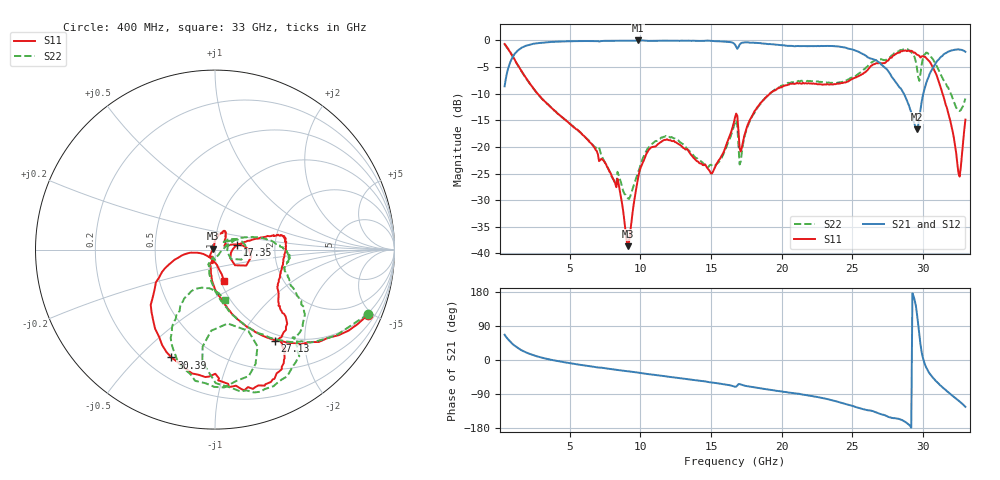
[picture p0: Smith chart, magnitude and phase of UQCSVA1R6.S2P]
!  Part Number  UQCSVA1R6  Mounting Orientation: Horizontal
!  Description: Ultra Low ESR Microwave capacitors
!  Application: Coupling, Bypass, Tuning, DC Block
!  Filters, Matching
# GHZ S DB R 50
! Freq  |S11|  S11 Ph  |S21|  S21 Ph  |S12|  S12 Ph  |S22|  S22 Ph
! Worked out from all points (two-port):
!   401 points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, 400 MHz to 33 GHz, reference 50 ohm
!   highest |S21| = 0.00 dB at 9.854 GHz (marker M1); lowest = -16.7 dB at 29.58 GHz (marker M2)
!   |S21| within 3 dB of the highest: 1 GHz to 26.02 GHz (25.02 GHz wide, 185 % of centre); 31.31 GHz to end of sweep
!   lowest |S11| = -38.6 dB at 9.121 GHz (marker M3), VSWR 1.02, Z = 48.9 + j0.482 ohm
!   |S11| at or under -10 dB: 2.737 GHz to 19.16 GHz (16.43 GHz wide, 150 % of centre); 31.38 GHz to end of sweep
!   |S22| runs from -29.8 to -0.7 dB; largest |S21 - S12| = 0.0079
!   S11 on the Smith chart (normalised r, x): 400 MHz: 0.92, -4.70; 17.35 GHz: 1.28, +0.06; 27.13 GHz: 0.89, -1.45; 30.39 GHz: 0.30, -0.63; 33 GHz: 1.04, -0.37
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0.4  -0.67 -23.2  -8.61 66.7  -8.61 66.5  -0.66 -22.9
2.193  -8.13 -73.2  -0.77 15.9  -0.78 16.0  -8.16 -73.6
5.861  -17.56 -100.0  -0.13 -13.3  -0.12 -13.4  -17.53 -104.0
8.387  -25.96 -128.3  -0.06 -26.4  -0.07 -26.6  -24.67 -91.6
9.121  -38.63 155.1  -0.05 -29.8  -0.06 -29.9  -29.63 -40.6
9.854  -25.68 88.7  0.00 -33.3  -0.01 -33.4  -24.67 14.7
11.321  -19.34 67.0  -0.06 -40.6  -0.06 -40.8  -18.56 26.9
15.07  -24.98 23.0  -0.12 -59.5  -0.12 -59.5  -23.48 38.7
16.7  -14.46 0.0  -0.77 -70.5  -0.77 -70.2  -15.41 9.0
17.108  -20.86 -10.9  -0.56 -64.6  -0.56 -64.7  -22.72 14.0
17.352  -17.94 11.0  -0.37 -67.4  -0.37 -67.4  -18.36 26.0
19.145  -10.05 13.7  -0.67 -78.4  -0.68 -78.3  -10.02 9.2
22.161  -8.13 0.6  -1.07 -95.1  -1.06 -95.0  -7.65 -8.0
27.132  -4.30 -56.9  -4.70 -144.4  -4.74 -144.3  -3.61 -48.1
27.621  -3.44 -55.5  -6.06 -151.0  -6.07 -151.0  -3.23 -48.6
28.925  -1.96 -73.6  -11.67 -168.2  -11.62 -168.0  -1.67 -74.8
29.577  -2.67 -87.2  -16.68 120.7  -16.82 120.5  -5.27 -97.3
29.985  -2.95 -94.3  -10.41 7.1  -10.48 6.5  -3.40 -70.5
30.392  -3.77 -112.0  -6.89 -31.3  -6.86 -30.9  -2.54 -94.0
31.452  -10.52 -159.5  -2.63 -74.5  -2.61 -74.2  -7.45 -120.5
32.511  -24.92 -143.5  -1.67 -106.8  -1.67 -107.0  -13.08 -104.1
33  -14.87 -74.1  -2.13 -123.6  -2.10 -123.6  -10.91 -79.1
